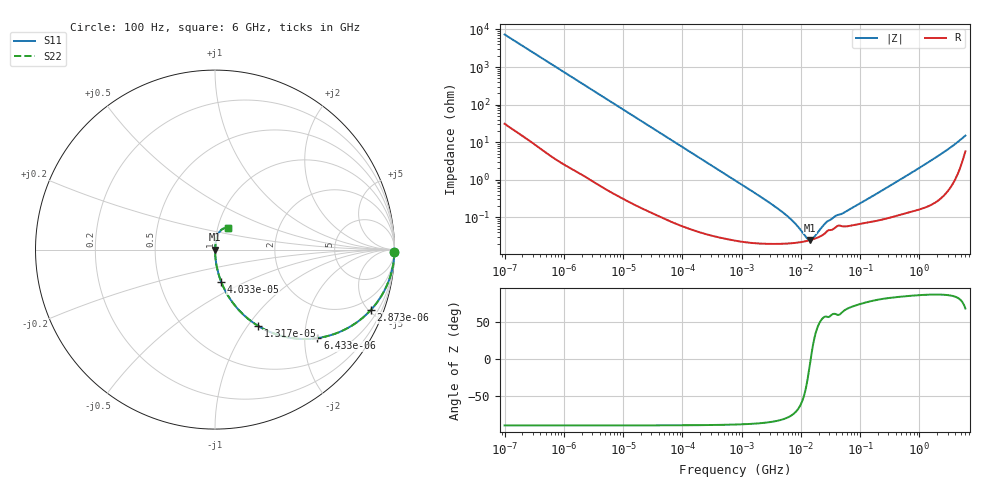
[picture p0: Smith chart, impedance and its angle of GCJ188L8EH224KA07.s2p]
!Murata Part Number: GCJ188L8EH224KA07
!These Parameters are Measured in Series Mode Connection
!Data Generated on Mar 13, 2026
!  o--ll--o
!Port1  Port2
!  o------o
!Operation Temp=25[degC], DC Bias Voltage=0[V]
!Freq. Start=100[Hz] Stop=6[GHz] 401[Steps]
# Hz S RI R 50
!Freq.(Hz) S11(Real) S11(Imag) S21(Real) S21(Imag) S12(Real) S12(Imag) S22(Real) S22(Imag)
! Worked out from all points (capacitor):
!   401 points, 100 Hz to 6 GHz, reference 50 ohm
!   read as one part in series: C = 216 nF near 109 Hz
!   lowest |Z| = 25 mohm at 14.22 MHz (marker M1)
!   series resonance near 14.73 MHz, so ESL is about 540 pH
!   S11 on the Smith chart (normalised r, x): 100 Hz: open; 2.873 kHz: 1.02, -5.15; 6.433 kHz: 1.01, -2.30; 13.17 kHz: 1.00, -1.13; 40.34 kHz: 1.00, -0.37; 6 GHz: 1.11, +0.28
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100  0.9998 -0.0136  0.000243 0.0136  0.000243 0.0136  0.9998 -0.0136
600  0.9932 -0.0807  0.00684 0.0807  0.00684 0.0807  0.9932 -0.0807
2008  0.9305 -0.2525  0.0695 0.2525  0.0695 0.2525  0.9305 -0.2525
2873  0.868 -0.3366  0.132 0.3366  0.132 0.3366  0.868 -0.3366
4299  0.7471 -0.4328  0.2529 0.4328  0.2529 0.4328  0.7471 -0.4328
6433  0.5701 -0.4931  0.4299 0.4931  0.4299 0.4931  0.5701 -0.4931
9204  0.3943 -0.4866  0.6057 0.4866  0.6057 0.4866  0.3943 -0.4866
13169  0.2422 -0.4262  0.7578 0.4262  0.7578 0.4262  0.2422 -0.4262
21550  0.1075 -0.3074  0.8925 0.3074  0.8925 0.3074  0.1075 -0.3074
40335  0.0339 -0.1782  0.9661 0.1782  0.9661 0.1782  0.0339 -0.1782
129199  0.00383 -0.0576  0.9962 0.0576  0.9962 0.0576  0.00383 -0.0576
774597  0.000334 -0.00969  0.9997 0.00969  0.9997 0.00969  0.000334 -0.00969
5079039  0.0002 -0.00131  0.9998 0.00131  0.9998 0.00131  0.0002 -0.00131
7947587  0.000209 -0.000668  0.9998 0.000668  0.9998 0.000668  0.000209 -0.000668
1.243624e7  0.000234 -0.000171  0.9998 0.000171  0.9998 0.000171  0.000234 -0.000171
1.422411e7  0.000247 -3.47e-05  0.9998 3.47e-05  0.9998 3.47e-05  0.000247 -3.47e-05
1.555665e7  0.000258 5.5e-05  0.9997 -5.5e-05  0.9997 -5.5e-05  0.000258 5.5e-05
2.434276e7  0.000353 0.000516  0.9996 -0.000516  0.9996 -0.000516  0.000353 0.000516
2.911731e7  0.000453 0.00067  0.9995 -0.00067  0.9995 -0.00067  0.000453 0.00067
3.124326e8  0.00102 0.0067  0.999 -0.0067  0.999 -0.0067  0.00102 0.0067
3.205649e9  0.0102 0.0672  0.9898 -0.0672  0.9898 -0.0672  0.0102 0.0672
6e9  0.0699 0.1215  0.9301 -0.1215  0.9301 -0.1215  0.0699 0.1215
